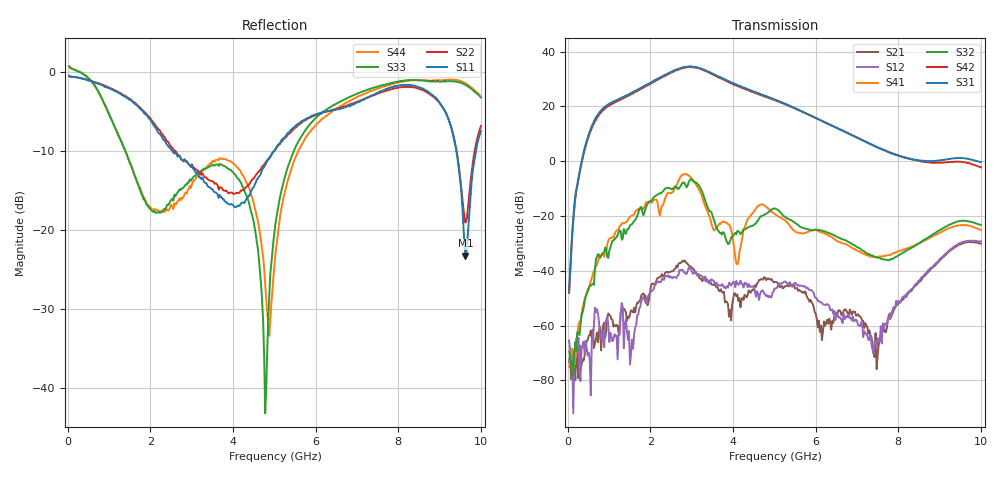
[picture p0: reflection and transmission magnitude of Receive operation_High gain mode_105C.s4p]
! Device:  ADRF5545A
! Description: Dual-Channel, Receiver Front End
! Frequency:  2.4 -  4.2 GHz
! Ports:
!	ANT-CHA	= Port 1
!	ANT-CHB	= Port 2
!  RXOUT-CHA = Port 3
!	RXOUT-CHB = Port 4
! VDD1-CHA, VDD1-CHB, VDD2-CHA, VDD2-CHB, and SWVDD-CHAB = 5 V
! SWCTRL-CHAB = 0 V,  PD-CHAB = 0 V,BP-CHA=BP-CHB=0V
! Temp=105C
! Data:  Data was collected using a calibrated 4 port network analyzer and de-embedded using AtaiTec's In Situ De-Embedding.
! Note:  Analog Devices supplies this data as a sample of measured data
!  for this product.  Your particular data for this product may vary.
!  Data was taken at 105 degrees C.
!  Analog Devices reserves the right to change this data at anytime.
!Correction: S11(Full 4 Port(1,2,3,4))
!S12(Full 4 Port(1,2,3,4))
!S13(Full 4 Port(1,2,3,4))
!S14(Full 4 Port(1,2,3,4))
!S21(Full 4 Port(1,2,3,4))
!S22(Full 4 Port(1,2,3,4))
!S23(Full 4 Port(1,2,3,4))
!S24(Full 4 Port(1,2,3,4))
!S31(Full 4 Port(1,2,3,4))
!S32(Full 4 Port(1,2,3,4))
!S33(Full 4 Port(1,2,3,4))
!S34(Full 4 Port(1,2,3,4))
!S41(Full 4 Port(1,2,3,4))
!S42(Full 4 Port(1,2,3,4))
!S43(Full 4 Port(1,2,3,4))
!S44(Full 4 Port(1,2,3,4))
!S4P File: Measurements: <S11,S12,S13,S14>,
!<S21,S22,S23,S24>,
!<S31,S32,S33,S34>,
!<S41,S42,S43,S44>:
# Hz S  dB  R 50
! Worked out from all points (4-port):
!   400 points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, 34.98 MHz to 10 GHz, reference 50 ohm
!   strongest paths, dB at 34.98 MHz, 2.532 GHz, 5.03 GHz, 7.527 GHz, 10 GHz:
!     S31: -47.4, 32.9, 22.4, 4.8, -0.4
!     S42: -48.0, 32.5, 22.2, 4.9, -2.2
!     S32: -69.4, -10.2, -17.3, -35.2, -23.3
!     S41: -75.1, -11.3, -19.5, -34.8, -25.1
!     S12: -65.5, -42.8, -46.5, -65.2, -29.3
!     S21: -73.2, -40.2, -44.0, -67.1, -30.1
!   lowest |S11| = -23.3 dB at 9.625 GHz (marker M1), VSWR 1.15, Z = 45.7 + j4.99 ohm
!   |S11| at or under -10 dB: 2.535 GHz to 5 GHz (2.465 GHz wide, 65.4 % of centre); 9.407 GHz to 9.883 GHz (476.1 MHz wide, 4.94 % of centre)
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3.4975e7  -0.48 -10.2  -65.52 47.3  -66.76 -133.9  -63.47 123.8
          -73.23 -46.6  -0.53 -10.0  -65.54 162.8  -63.51 -152.1
          -47.42 -107.1  -69.44 -90.5  0.68 -9.8  -61.01 -18.9
          -75.12 30.8  -48.04 -113.8  -65.18 8.8  0.72 -9.8
1.85815e9  -5.27 -130.2  -50.20 173.5  -60.78 88.3  -74.12 124.7
           -49.21 161.2  -5.09 -129.1  -67.74 107.9  -61.12 90.5
           27.44 -47.9  -18.55 -40.8  -16.17 139.0  -59.76 -138.1
           -16.58 -56.5  27.07 -44.4  -50.42 -171.1  -15.97 133.5
2.882125e9  -11.30 83.3  -41.01 66.4  -57.69 32.2  -80.12 15.0
            -37.12 40.8  -11.35 91.5  -74.36 105.4  -58.36 33.2
            34.56 173.2  -9.49 95.7  -14.26 -6.1  -46.87 130.6
            -4.77 90.5  34.24 177.2  -48.97 172.4  -15.40 -9.6
3.3067e9  -13.99 4.5  -42.30 20.8  -56.96 17.4  -65.80 73.5
          -43.14 0.3  -13.27 13.0  -74.88 92.9  -58.12 14.7
          33.41 104.0  -13.27 -57.8  -12.26 -31.3  -54.72 86.7
          -15.46 -64.3  33.17 106.9  -48.83 103.3  -12.28 -39.7
3.881125e9  -16.69 -35.2  -46.10 21.4  -57.90 -2.2  -74.03 -56.7
            -52.31 -20.2  -15.34 -16.1  -71.89 78.3  -58.81 -3.9
            29.36 33.2  -30.24 78.5  -12.27 -49.7  -47.34 116.9
            -22.99 -8.0  29.02 37.0  -51.16 73.7  -11.22 -54.0
9.625375e9  -23.27 127.6  -29.26 -110.6  -61.02 30.5  -65.94 -0.9
            -29.68 -116.2  -19.09 138.9  -65.54 14.3  -64.28 132.2
            1.03 -21.5  -21.77 -71.2  -1.64 103.6  -61.13 62.2
            -23.31 -69.7  -0.44 -18.9  -66.12 16.9  -1.43 98.4
1e10  -7.49 -149.6  -29.27 -171.8  -65.29 113.2  -64.20 58.3
      -30.07 -178.0  -6.84 -156.7  -65.40 11.7  -62.29 140.0
      -0.35 -64.3  -23.27 -136.7  -3.23 105.0  -58.87 71.7
      -25.10 -134.3  -2.25 -60.3  -63.76 53.7  -3.11 101.5
